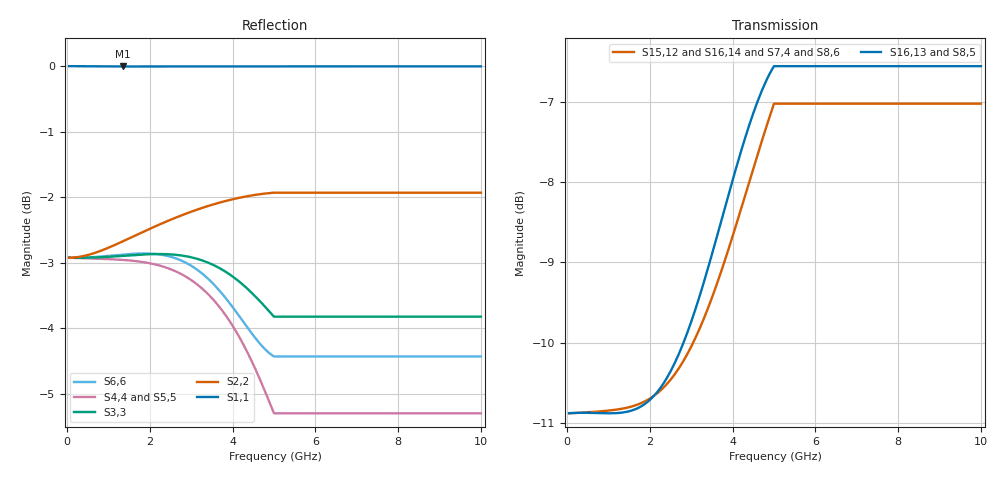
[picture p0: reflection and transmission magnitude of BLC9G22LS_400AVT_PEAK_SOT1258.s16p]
! Created Tue Apr 19 12:43:08 2016
! 16 Port Network Data from SP1.SP block
! freq  magS1_1  angS1_1  magS1_2  angS1_2  magS1_3  angS1_3  magS1_4  angS1_4
!  magS1_5  angS1_5  magS1_6  angS1_6  magS1_7  angS1_7  magS1_8  angS1_8
!  magS1_9  angS1_9  magS1_10  angS1_10  magS1_11  angS1_11  magS1_12  angS1_12
!  magS1_13  angS1_13  magS1_14  angS1_14  magS1_15  angS1_15  magS1_16  angS1_16
!  magS2_1  angS2_1  magS2_2  angS2_2  magS2_3  angS2_3  magS2_4  angS2_4
!  magS2_5  angS2_5  magS2_6  angS2_6  magS2_7  angS2_7  magS2_8  angS2_8
!  magS2_9  angS2_9  magS2_10  angS2_10  magS2_11  angS2_11  magS2_12  angS2_12
!  magS2_13  angS2_13  magS2_14  angS2_14  magS2_15  angS2_15  magS2_16  angS2_16
!  magS3_1  angS3_1  magS3_2  angS3_2  magS3_3  angS3_3  magS3_4  angS3_4
!  magS3_5  angS3_5  magS3_6  angS3_6  magS3_7  angS3_7  magS3_8  angS3_8
!  magS3_9  angS3_9  magS3_10  angS3_10  magS3_11  angS3_11  magS3_12  angS3_12
!  magS3_13  angS3_13  magS3_14  angS3_14  magS3_15  angS3_15  magS3_16  angS3_16
!  magS4_1  angS4_1  magS4_2  angS4_2  magS4_3  angS4_3  magS4_4  angS4_4
!  magS4_5  angS4_5  magS4_6  angS4_6  magS4_7  angS4_7  magS4_8  angS4_8
!  magS4_9  angS4_9  magS4_10  angS4_10  magS4_11  angS4_11  magS4_12  angS4_12
!  magS4_13  angS4_13  magS4_14  angS4_14  magS4_15  angS4_15  magS4_16  angS4_16
!  magS5_1  angS5_1  magS5_2  angS5_2  magS5_3  angS5_3  magS5_4  angS5_4
!  magS5_5  angS5_5  magS5_6  angS5_6  magS5_7  angS5_7  magS5_8  angS5_8
!  magS5_9  angS5_9  magS5_10  angS5_10  magS5_11  angS5_11  magS5_12  angS5_12
!  magS5_13  angS5_13  magS5_14  angS5_14  magS5_15  angS5_15  magS5_16  angS5_16
!  magS6_1  angS6_1  magS6_2  angS6_2  magS6_3  angS6_3  magS6_4  angS6_4
!  magS6_5  angS6_5  magS6_6  angS6_6  magS6_7  angS6_7  magS6_8  angS6_8
!  magS6_9  angS6_9  magS6_10  angS6_10  magS6_11  angS6_11  magS6_12  angS6_12
!  magS6_13  angS6_13  magS6_14  angS6_14  magS6_15  angS6_15  magS6_16  angS6_16
!  magS7_1  angS7_1  magS7_2  angS7_2  magS7_3  angS7_3  magS7_4  angS7_4
!  magS7_5  angS7_5  magS7_6  angS7_6  magS7_7  angS7_7  magS7_8  angS7_8
!  magS7_9  angS7_9  magS7_10  angS7_10  magS7_11  angS7_11  magS7_12  angS7_12
!  magS7_13  angS7_13  magS7_14  angS7_14  magS7_15  angS7_15  magS7_16  angS7_16
!  magS8_1  angS8_1  magS8_2  angS8_2  magS8_3  angS8_3  magS8_4  angS8_4
!  magS8_5  angS8_5  magS8_6  angS8_6  magS8_7  angS8_7  magS8_8  angS8_8
!  magS8_9  angS8_9  magS8_10  angS8_10  magS8_11  angS8_11  magS8_12  angS8_12
!  magS8_13  angS8_13  magS8_14  angS8_14  magS8_15  angS8_15  magS8_16  angS8_16
!  magS9_1  angS9_1  magS9_2  angS9_2  magS9_3  angS9_3  magS9_4  angS9_4
!  magS9_5  angS9_5  magS9_6  angS9_6  magS9_7  angS9_7  magS9_8  angS9_8
!  magS9_9  angS9_9  magS9_10  angS9_10  magS9_11  angS9_11  magS9_12  angS9_12
!  magS9_13  angS9_13  magS9_14  angS9_14  magS9_15  angS9_15  magS9_16  angS9_16
!  magS10_1  angS10_1  magS10_2  angS10_2  magS10_3  angS10_3  magS10_4  angS10_4
!  magS10_5  angS10_5  magS10_6  angS10_6  magS10_7  angS10_7  magS10_8  angS10_8
!  magS10_9  angS10_9  magS10_10  angS10_10  magS10_11  angS10_11  magS10_12  angS10_12
!  magS10_13  angS10_13  magS10_14  angS10_14  magS10_15  angS10_15  magS10_16  angS10_16
!  magS11_1  angS11_1  magS11_2  angS11_2  magS11_3  angS11_3  magS11_4  angS11_4
!  magS11_5  angS11_5  magS11_6  angS11_6  magS11_7  angS11_7  magS11_8  angS11_8
!  magS11_9  angS11_9  magS11_10  angS11_10  magS11_11  angS11_11  magS11_12  angS11_12
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# ghz S ma R 50
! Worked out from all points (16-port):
!   200 points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, 50 MHz to 10 GHz, reference 50 ohm
!   strongest paths, dB at 50 MHz, 2.55 GHz, 5.05 GHz, 7.55 GHz, 10 GHz:
!     S16,13: -10.9, -10.3, -6.6, -6.6, -6.6
!     S8,5: -10.9, -10.3, -6.6, -6.6, -6.6
!     S15,12: -10.9, -10.4, -7.0, -7.0, -7.0
!     S16,14: -10.9, -10.7, -7.1, -7.1, -7.1
!     S7,4: -10.9, -10.4, -7.1, -7.1, -7.1
!     S8,6: -10.9, -10.7, -7.1, -7.1, -7.1
!   lowest |S11| = 0.0 dB at 1.35 GHz (marker M1)
!   |S11| at or under -10 dB: nowhere
